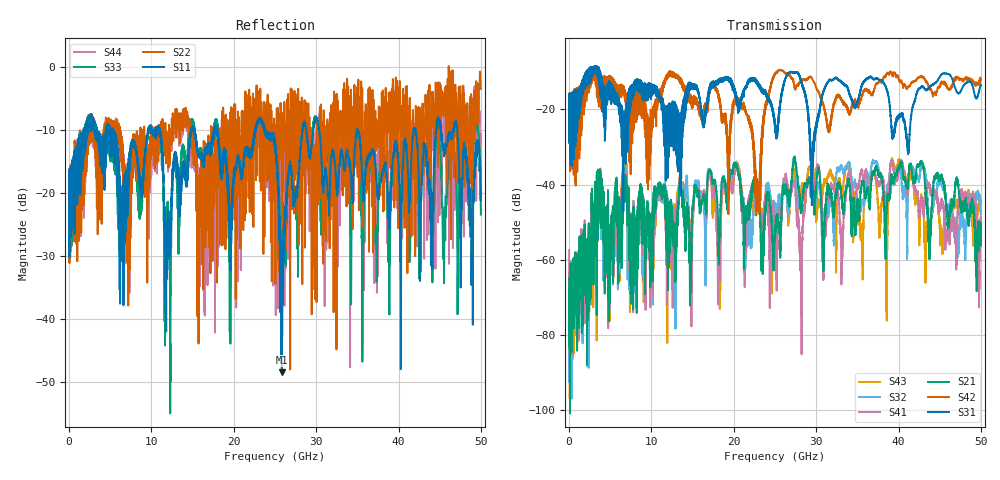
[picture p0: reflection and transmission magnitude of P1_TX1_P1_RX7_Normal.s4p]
!Keysight Technologies,N5225B,MY57041031,A.13.20.10
!Date: Friday, May 31, 2019 11:23:53
!Correction: S11(Full 4 Port(1,2,3,4))
!S12(Full 4 Port(1,2,3,4))
!S13(Full 4 Port(1,2,3,4))
!S14(Full 4 Port(1,2,3,4))
!S21(Full 4 Port(1,2,3,4))
!S22(Full 4 Port(1,2,3,4))
!S23(Full 4 Port(1,2,3,4))
!S24(Full 4 Port(1,2,3,4))
!S31(Full 4 Port(1,2,3,4))
!S32(Full 4 Port(1,2,3,4))
!S33(Full 4 Port(1,2,3,4))
!S34(Full 4 Port(1,2,3,4))
!S41(Full 4 Port(1,2,3,4))
!S42(Full 4 Port(1,2,3,4))
!S43(Full 4 Port(1,2,3,4))
!S44(Full 4 Port(1,2,3,4))
!S4P File: Measurements: <S11,S12,S13,S14>,
!<S21,S22,S23,S24>,
!<S31,S32,S33,S34>,
!<S41,S42,S43,S44>:
# Hz S  dB  R 50.0
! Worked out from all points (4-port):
!   5000 points, 10 MHz to 50 GHz, reference 50 ohm
!   strongest paths, dB at 10 MHz, 12.51 GHz, 25.01 GHz, 37.51 GHz, 50 GHz:
!     S31: -19.3, -29.2, -24.6, -11.8, -13.5
!     S42: -19.6, -10.0, -10.7, -12.9, -12.2
!     S21: -64.9, -47.9, -53.0, -36.8, -53.2
!     S41: -57.4, -50.8, -50.9, -39.7, -49.7
!     S32: -69.7, -49.1, -46.3, -35.2, -48.1
!     S43: -64.5, -47.5, -52.5, -45.4, -45.2
!   lowest |S11| = -48.4 dB at 25.83 GHz (marker M1), VSWR 1.01, Z = 49.9 + j0.374 ohm
!   |S11| at or under -10 dB: 18.01 GHz to 22.61 GHz (4.596 GHz wide, 22.6 % of centre); 30.38 GHz to 34.94 GHz (4.561 GHz wide, 14 % of centre); 34.98 GHz to 41.81 GHz (6.835 GHz wide, 17.8 % of centre)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
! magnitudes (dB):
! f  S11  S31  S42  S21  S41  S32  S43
! 10 MHz  -19.9  -19.3  -19.6  -64.9  -57.4  -69.7  -64.5
! 3.62 GHz  -11.9  -12.2  -19.3  -46.2  -47.1  -45.8  -46.5
! 20.5 GHz  -14.0  -18.6  -17.1  -36.7  -36.6  -36.1  -34.8
! 22.93 GHz  -8.7  -13.4  -39.8  -40.1  -40.3  -42.8  -43.4
! 25.83 GHz  -48.4  -16.0  -9.6  -45.2  -46.3  -47.5  -46.3
! 28.56 GHz  -8.6  -15.0  -12.2  -40.2  -47.8  -40.7  -42.7
! 50 GHz  -19.8  -13.5  -12.2  -53.2  -49.7  -48.1  -45.2
